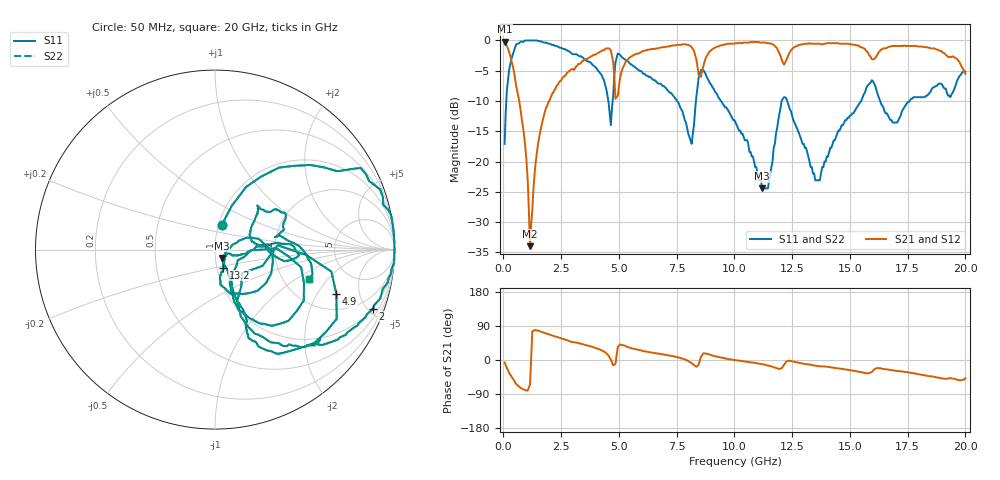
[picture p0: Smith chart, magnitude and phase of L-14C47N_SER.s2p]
# MHZ S MA R 50
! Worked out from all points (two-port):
!   400 points, 50 MHz to 20 GHz, reference 50 ohm
!   highest |S21| = -0.18 dB at 50 MHz (marker M1); lowest = -34.0 dB at 1.15 GHz (marker M2)
!   |S21| within 3 dB of the highest: 8.734 GHz to 12.05 GHz (3.312 GHz wide, 31.9 % of centre); 12.25 GHz to 19.67 GHz (7.411 GHz wide, 46.4 % of centre)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
!   lowest |S11| = -24.4 dB at 11.2 GHz (marker M3), VSWR 1.13, Z = 53.8 - j4.96 ohm
!   |S11| at or under -10 dB: 9.419 GHz to 12.05 GHz (2.627 GHz wide, 24.5 % of centre); 12.28 GHz to 15.48 GHz (3.197 GHz wide, 23 % of centre); 16.31 GHz to 17.58 GHz (1.272 GHz wide, 7.51 % of centre)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
!   |S22| runs from -24.4 to 0.0 dB; largest |S21 - S12| = 0
!   S11 on the Smith chart (normalised r, x): 50 MHz: 1.04, +0.29; 2 GHz: 0.95, -5.37; 4.9 GHz: 2.90, -2.98; 13.2 GHz: 1.07, -0.22; 20 GHz: 2.77, -1.29
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50  0.14 74.7  0.98 -6.5  0.98 -6.5  0.14 74.7
250  0.58 52.0  0.8 -33.8  0.8 -33.8  0.58 52.0
900  0.99 13.0  0.16 -78.6  0.16 -78.6  0.99 13.0
1150  1 4.3  0.02 -64.9  0.02 -64.9  1 4.3
1450  1 -4.4  0.12 78.4  0.12 78.4  1 -4.4
2000  0.94 -20.5  0.32 67.0  0.32 67.0  0.94 -20.5
3400  0.73 -48.0  0.67 42.1  0.67 42.1  0.73 -48.0
4650  0.2 -41.5  0.83 0.7  0.83 0.7  0.2 -41.5
4900  0.72 -20.1  0.34 12.4  0.34 12.4  0.72 -20.1
5350  0.68 -58.6  0.69 34.8  0.69 34.8  0.68 -58.6
6700  0.44 -67.0  0.86 16.8  0.86 16.8  0.44 -67.0
8150  0.14 -25.2  0.88 -8.4  0.88 -8.4  0.14 -25.2
8550  0.57 -29.8  0.5 8.4  0.5 8.4  0.57 -29.8
10050  0.21 -67.0  0.95 -0.4  0.95 -0.4  0.21 -67.0
11200  0.06 -50.0  0.96 -11.0  0.96 -11.0  0.06 -50.0
12150  0.34 -22.9  0.63 -12.4  0.63 -12.4  0.34 -22.9
13200  0.11 -65.7  0.94 -11.7  0.94 -11.7  0.11 -65.7
13350  0.09 -55.1  0.94 -13.4  0.94 -13.4  0.09 -55.1
15950  0.47 -3.6  0.7 -31.5  0.7 -31.5  0.47 -3.6
16700  0.23 8.2  0.89 -25.8  0.89 -25.8  0.23 8.2
18600  0.41 33.3  0.86 -43.9  0.86 -43.9  0.41 33.3
20000  0.55 -17.2  0.53 -48.0  0.53 -48.0  0.55 -17.2
